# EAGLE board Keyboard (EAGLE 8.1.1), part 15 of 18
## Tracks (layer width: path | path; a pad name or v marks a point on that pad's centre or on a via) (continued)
S$15455 (continued)
  Bottom 0: 222.84,60.24 222.79,60.14
S$15456
  Bottom 0: 222.79,60.14 222.71,59.8
S$15457
  Bottom 0: 222.71,59.8 222.71,59.45
S$15458
  Bottom 0: 222.71,59.45 222.79,59.11
S$15459
  Bottom 0: 222.79,59.11 222.96,58.8
S$15460
  Bottom 0: 222.96,58.8 223.2,58.55
S$15461
  Bottom 0: 223.2,58.55 223.5,58.36
S$15462
  Bottom 0: 223.5,58.36 223.83,58.26
S$15463
  Bottom 0: 223.83,58.26 224.18,58.23
S$15464
  Bottom 0: 224.18,58.23 224.52,58.3
S$15465
  Bottom 0: 224.52,58.3 224.84,58.45
S$15466
  Bottom 0: 224.84,58.45 225.11,58.67
S$15467
  Bottom 0: 225.11,58.67 225.32,58.96
S$15468
  Bottom 0: 225.32,58.96 225.44,59.28
S$15469
  Bottom 0: 225.44,59.28 225.49,59.63
S$15470
  Bottom 0: 225.49,59.63 225.44,59.97
S$15471
  Bottom 0: 225.44,59.97 225.32,60.3
S$15472
  Bottom 0: 225.32,60.3 225.11,60.58
S$15473
  Bottom 0: 225.11,60.58 224.84,60.8
S$15474
  Bottom 0: 224.84,60.8 224.52,60.96
S$15475
  Bottom 0: 224.52,60.96 224.18,61.02
S$15476
  Bottom 0: 224.18,61.02 223.83,61
S$15477
  Bottom 0: 223.83,61 223.5,60.89
S$15478
  Bottom 0: 223.5,60.89 223.47,60.87
S$15479
  Bottom 0: 223.47,60.87 222.89,61.45
S$15480
  Bottom 0: 222.89,61.45 222.84,61.48
S$15481
  Bottom 0: 222.84,61.48 222.78,61.53
S$15482
  Bottom 0: 222.78,61.53 222.72,61.55
S$15483
  Bottom 0: 222.72,61.55 222.65,61.57
S$15484
  Bottom 0: 222.65,61.57 222.58,61.57
S$15485
  Bottom 0: 222.58,61.57 218.02,61.57
S$15486
  Bottom 0: 218.02,61.57 217.96,61.7
S$15487
  Bottom 0: 217.96,61.7 217.94,61.73
S$15488
  Bottom 0: 217.94,61.73 229.12,61.73
S$15489
  Bottom 0: 229.12,61.73 229.14,61.65
S$15490
  Bottom 0: 229.14,61.65 229.31,61.34
S$15491
  Bottom 0: 229.31,61.34 229.55,61.09
S$15492
  Bottom 0: 229.55,61.09 229.85,60.9
S$15493
  Bottom 0: 229.85,60.9 230.18,60.8
S$15494
  Bottom 0: 230.18,60.8 230.53,60.77
S$15495
  Bottom 0: 230.53,60.77 230.87,60.84
S$15496
  Bottom 0: 230.87,60.84 231.19,60.99
S$15497
  Bottom 0: 231.19,60.99 231.46,61.21
S$15498
  Bottom 0: 231.46,61.21 231.67,61.5
S$15499
  Bottom 0: 231.67,61.5 231.76,61.73
S$15500
  Bottom 0: 231.76,61.73 231.79,61.73
S$15501
  Bottom 0: 231.79,61.73 241.11,52.41
S$15502
  Bottom 0: 227.53,52.8 227.85,52.82
S$15503
  Bottom 0: 227.85,52.82 228.16,52.93
S$15504
  Bottom 0: 228.16,52.93 228.42,53.11
S$15505
  Bottom 0: 228.42,53.11 228.62,53.37
S$15506
  Bottom 0: 228.62,53.37 228.75,53.67
S$15507
  Bottom 0: 228.75,53.67 228.8,53.98
S$15508
  Bottom 0: 228.8,53.98 228.75,54.3
S$15509
  Bottom 0: 228.75,54.3 228.62,54.61
S$15510
  Bottom 0: 228.62,54.61 228.42,54.86
S$15511
  Bottom 0: 228.42,54.86 228.16,55.05
S$15512
  Bottom 0: 228.16,55.05 227.85,55.16
S$15513
  Bottom 0: 227.85,55.16 227.53,55.18
S$15514
  Bottom 0: 227.53,55.18 227.21,55.11
S$15515
  Bottom 0: 227.21,55.11 226.91,54.96
S$15516
  Bottom 0: 226.91,54.96 226.68,54.74
S$15517
  Bottom 0: 226.68,54.74 226.51,54.47
S$15518
  Bottom 0: 226.51,54.47 226.42,54.15
S$15519
  Bottom 0: 226.42,54.15 226.42,53.83
S$15520
  Bottom 0: 226.42,53.83 226.51,53.51
S$15521
  Bottom 0: 226.51,53.51 226.68,53.23
S$15522
  Bottom 0: 226.68,53.23 226.91,53.01
S$15523
  Bottom 0: 226.91,53.01 227.21,52.87
S$15524
  Bottom 0: 227.21,52.87 227.53,52.8
S$15525
  Bottom 0: 235.15,52.8 235.47,52.82
S$15526
  Bottom 0: 235.47,52.82 235.78,52.93
S$15527
  Bottom 0: 235.78,52.93 236.04,53.11
S$15528
  Bottom 0: 236.04,53.11 236.25,53.37
S$15529
  Bottom 0: 236.25,53.37 236.37,53.67
S$15530
  Bottom 0: 236.37,53.67 236.42,53.98
S$15531
  Bottom 0: 236.42,53.98 236.37,54.3
S$15532
  Bottom 0: 236.37,54.3 236.25,54.61
S$15533
  Bottom 0: 236.25,54.61 236.04,54.86
S$15534
  Bottom 0: 236.04,54.86 235.78,55.05
S$15535
  Bottom 0: 235.78,55.05 235.47,55.16
S$15536
  Bottom 0: 235.47,55.16 235.15,55.18
S$15537
  Bottom 0: 235.15,55.18 234.83,55.11
S$15538
  Bottom 0: 234.83,55.11 234.53,54.96
S$15539
  Bottom 0: 234.53,54.96 234.3,54.74
S$15540
  Bottom 0: 234.3,54.74 234.13,54.47
S$15541
  Bottom 0: 234.13,54.47 234.04,54.15
S$15542
  Bottom 0: 234.04,54.15 234.04,53.83
S$15543
  Bottom 0: 234.04,53.83 234.13,53.51
S$15544
  Bottom 0: 234.13,53.51 234.3,53.23
S$15545
  Bottom 0: 234.3,53.23 234.53,53.01
S$15546
  Bottom 0: 234.53,53.01 234.83,52.87
S$15547
  Bottom 0: 234.83,52.87 235.15,52.8
S$15548
  Bottom 0: 103.73,52.93 103,53.65
S$15549
  Bottom 0: 103,53.65 103.01,53.67
S$15550
  Bottom 0: 103.01,53.67 103.06,53.98
S$15551
  Bottom 0: 103.06,53.98 103.01,54.3
S$15552
  Bottom 0: 103.01,54.3 103,54.33
S$15553
  Bottom 0: 103,54.33 104.49,55.82
S$15554
  Bottom 0: 104.49,55.82 104.55,55.88
S$15555
  Bottom 0: 104.55,55.88 104.6,55.96
S$15556
  Bottom 0: 104.6,55.96 104.64,56.04
S$15557
  Bottom 0: 104.64,56.04 104.66,56.13
S$15558
  Bottom 0: 104.66,56.13 104.66,56.22
S$15559
  Bottom 0: 104.66,56.22 104.66,72.65
S$15560
  Bottom 0: 104.66,72.65 104.97,72.95
S$15561
  Bottom 0: 104.97,72.95 104.97,72.9
S$15562
  Bottom 0: 104.97,72.9 105.06,72.67
S$15563
  Bottom 0: 105.06,72.67 105.23,72.48
S$15564
  Bottom 0: 105.23,72.48 105.45,72.37
S$15565
  Bottom 0: 105.45,72.37 105.48,72.37
S$15566
  Bottom 0: 105.48,72.37 110.3,67.55
S$15567
  Bottom 0: 110.3,67.55 110.36,67.51
S$15568
  Bottom 0: 110.36,67.51 110.42,67.47
S$15569
  Bottom 0: 110.42,67.47 110.48,67.44
S$15570
  Bottom 0: 110.48,67.44 110.54,67.42
S$15571
  Bottom 0: 110.54,67.42 110.61,67.42
S$15572
  Bottom 0: 110.61,67.42 112.51,67.42
S$15573
  Bottom 0: 112.51,67.42 113.08,66.86
S$15574
  Bottom 0: 113.08,66.86 112.78,66.94
S$15575
  Bottom 0: 112.78,66.94 112.33,66.99
S$15576
  Bottom 0: 112.33,66.99 111.88,66.94
S$15577
  Bottom 0: 111.88,66.94 111.45,66.82
S$15578
  Bottom 0: 111.45,66.82 111.06,66.61
S$15579
  Bottom 0: 111.06,66.61 110.72,66.32
S$15580
  Bottom 0: 110.72,66.32 110.43,65.98
S$15581
  Bottom 0: 110.43,65.98 110.22,65.58
S$15582
  Bottom 0: 110.22,65.58 110.09,65.15
S$15583
  Bottom 0: 110.09,65.15 110.05,64.71
S$15584
  Bottom 0: 110.05,64.71 110.09,64.26
S$15585
  Bottom 0: 110.09,64.26 110.22,63.83
S$15586
  Bottom 0: 110.22,63.83 110.43,63.44
S$15587
  Bottom 0: 110.43,63.44 110.72,63.09
S$15588
  Bottom 0: 110.72,63.09 111.06,62.81
S$15589
  Bottom 0: 111.06,62.81 111.45,62.59
S$15590
  Bottom 0: 111.45,62.59 111.88,62.47
S$15591
  Bottom 0: 111.88,62.47 112.33,62.42
S$15592
  Bottom 0: 112.33,62.42 112.78,62.47
S$15593
  Bottom 0: 112.78,62.47 113.2,62.59
S$15594
  Bottom 0: 113.2,62.59 113.6,62.81
S$15595
  Bottom 0: 113.6,62.81 113.95,63.09
S$15596
  Bottom 0: 113.95,63.09 114.23,63.44
S$15597
  Bottom 0: 114.23,63.44 114.44,63.83
S$15598
  Bottom 0: 114.44,63.83 114.57,64.26
S$15599
  Bottom 0: 114.57,64.26 114.62,64.71
S$15600
  Bottom 0: 114.62,64.71 114.57,65.15
S$15601
  Bottom 0: 114.57,65.15 114.48,65.45
S$15602
  Bottom 0: 114.48,65.45 115.7,64.24
S$15603
  Bottom 0: 115.7,64.24 115.7,63.48
S$15604
  Bottom 0: 115.7,63.48 115.55,63.43
S$15605
  Bottom 0: 115.55,63.43 115.25,63.24
S$15606
  Bottom 0: 115.25,63.24 115.01,62.99
S$15607
  Bottom 0: 115.01,62.99 114.84,62.68
S$15608
  Bottom 0: 114.84,62.68 114.75,62.34
S$15609
  Bottom 0: 114.75,62.34 114.75,61.99
S$15610
  Bottom 0: 114.75,61.99 114.84,61.65
S$15611
  Bottom 0: 114.84,61.65 115.01,61.34
S$15612
  Bottom 0: 115.01,61.34 115.25,61.09
S$15613
  Bottom 0: 115.25,61.09 115.55,60.9
S$15614
  Bottom 0: 115.55,60.9 115.88,60.8
S$15615
  Bottom 0: 115.88,60.8 116.23,60.77
S$15616
  Bottom 0: 116.23,60.77 116.57,60.84
S$15617
  Bottom 0: 116.57,60.84 116.75,60.93
S$15618
  Bottom 0: 116.75,60.93 121.83,55.85
S$15619
  Bottom 0: 121.83,55.85 121.83,54.74
S$15620
  Bottom 0: 121.83,54.74 121.73,54.87
S$15621
  Bottom 0: 121.73,54.87 121.47,55.05
S$15622
  Bottom 0: 121.47,55.05 121.16,55.16
S$15623
  Bottom 0: 121.16,55.16 120.83,55.18
S$15624
  Bottom 0: 120.83,55.18 120.52,55.12
S$15625
  Bottom 0: 120.52,55.12 120.23,54.97
S$15626
  Bottom 0: 120.23,54.97 119.99,54.74
S$15627
  Bottom 0: 119.99,54.74 119.82,54.47
S$15628
  Bottom 0: 119.82,54.47 119.73,54.16
S$15629
  Bottom 0: 119.73,54.16 119.73,53.83
S$15630
  Bottom 0: 119.73,53.83 119.78,53.66
S$15631
  Bottom 0: 119.78,53.66 119.04,52.93
S$15632
  Bottom 0: 119.04,52.93 113.83,52.93
S$15633
  Bottom 0: 113.83,52.93 113.84,52.93
S$15634
  Bottom 0: 113.84,52.93 114.11,53.12
S$15635
  Bottom 0: 114.11,53.12 114.32,53.37
S$15636
  Bottom 0: 114.32,53.37 114.44,53.67
S$15637
  Bottom 0: 114.44,53.67 114.49,53.99
S$15638
  Bottom 0: 114.49,53.99 114.44,54.31
S$15639
  Bottom 0: 114.44,54.31 114.32,54.61
S$15640
  Bottom 0: 114.32,54.61 114.11,54.87
S$15641
  Bottom 0: 114.11,54.87 113.84,55.05
S$15642
  Bottom 0: 113.84,55.05 113.54,55.16
S$15643
  Bottom 0: 113.54,55.16 113.22,55.18
S$15644
  Bottom 0: 113.22,55.18 112.89,55.12
S$15645
  Bottom 0: 112.89,55.12 112.61,54.97
S$15646
  Bottom 0: 112.61,54.97 112.37,54.74
S$15647
  Bottom 0: 112.37,54.74 112.2,54.47
S$15648
  Bottom 0: 112.2,54.47 112.11,54.16
S$15649
  Bottom 0: 112.11,54.16 112.11,53.83
S$15650
  Bottom 0: 112.11,53.83 112.2,53.52
S$15651
  Bottom 0: 112.2,53.52 112.37,53.24
S$15652
  Bottom 0: 112.37,53.24 112.61,53.02
S$15653
  Bottom 0: 112.61,53.02 112.78,52.93
S$15654
  Bottom 0: 112.78,52.93 103.73,52.93
S$15655
  Bottom 0: 109.88,58.23 110.22,58.3
S$15656
  Bottom 0: 110.22,58.3 110.54,58.45
S$15657
  Bottom 0: 110.54,58.45 110.81,58.67
S$15658
  Bottom 0: 110.81,58.67 111.02,58.96
S$15659
  Bottom 0: 111.02,58.96 111.14,59.28
S$15660
  Bottom 0: 111.14,59.28 111.19,59.63
S$15661
  Bottom 0: 111.19,59.63 111.14,59.97
S$15662
  Bottom 0: 111.14,59.97 111.02,60.3
S$15663
  Bottom 0: 111.02,60.3 110.81,60.58
S$15664
  Bottom 0: 110.81,60.58 110.54,60.8
S$15665
  Bottom 0: 110.54,60.8 110.22,60.96
S$15666
  Bottom 0: 110.22,60.96 109.88,61.02
S$15667
  Bottom 0: 109.88,61.02 109.53,61
S$15668
  Bottom 0: 109.53,61 109.2,60.89
S$15669
  Bottom 0: 109.2,60.89 108.9,60.7
S$15670
  Bottom 0: 108.9,60.7 108.66,60.45
S$15671
  Bottom 0: 108.66,60.45 108.49,60.14
S$15672
  Bottom 0: 108.49,60.14 108.41,59.8
S$15673
  Bottom 0: 108.41,59.8 108.41,59.45
S$15674
  Bottom 0: 108.41,59.45 108.49,59.11
S$15675
  Bottom 0: 108.49,59.11 108.66,58.8
S$15676
  Bottom 0: 108.66,58.8 108.9,58.55
S$15677
  Bottom 0: 108.9,58.55 109.2,58.36
S$15678
  Bottom 0: 109.2,58.36 109.53,58.26
S$15679
  Bottom 0: 109.53,58.26 109.88,58.23
S$15680
  Bottom 0: 262.06,52.98 258.88,56.16
S$15681
  Bottom 0: 258.88,56.16 258.87,56.17
S$15682
  Bottom 0: 258.87,56.17 253.59,61.45
S$15683
  Bottom 0: 253.59,61.45 253.53,61.5
S$15684
  Bottom 0: 253.53,61.5 253.48,61.54
S$15685
  Bottom 0: 253.48,61.54 253.41,61.56
S$15686
  Bottom 0: 253.41,61.56 253.35,61.58
S$15687
  Bottom 0: 253.35,61.58 253.28,61.58
S$15688
  Bottom 0: 253.28,61.58 250.75,61.58
S$15689
  Bottom 0: 250.75,61.58 250.84,61.82
S$15690
  Bottom 0: 250.84,61.82 250.89,62.17
S$15691
  Bottom 0: 250.89,62.17 250.84,62.51
S$15692
  Bottom 0: 250.84,62.51 250.72,62.84
S$15693
  Bottom 0: 250.72,62.84 250.51,63.12
S$15694
  Bottom 0: 250.51,63.12 250.24,63.34
S$15695
  Bottom 0: 250.24,63.34 249.92,63.5
S$15696
  Bottom 0: 249.92,63.5 249.57,63.56
S$15697
  Bottom 0: 249.57,63.56 249.23,63.54
S$15698
  Bottom 0: 249.23,63.54 248.9,63.43
S$15699
  Bottom 0: 248.9,63.43 248.6,63.24
S$15700
  Bottom 0: 248.6,63.24 248.36,62.99
S$15701
  Bottom 0: 248.36,62.99 248.19,62.68
S$15702
  Bottom 0: 248.19,62.68 248.17,62.61
S$15703
  Bottom 0: 248.17,62.61 246.59,62.61
S$15704
  Bottom 0: 246.59,62.61 246.95,62.81
S$15705
  Bottom 0: 246.95,62.81 247.29,63.09
S$15706
  Bottom 0: 247.29,63.09 247.58,63.44
S$15707
  Bottom 0: 247.58,63.44 247.79,63.83
S$15708
  Bottom 0: 247.79,63.83 247.92,64.26
S$15709
  Bottom 0: 247.92,64.26 247.97,64.71
S$15710
  Bottom 0: 247.97,64.71 247.92,65.15
S$15711
  Bottom 0: 247.92,65.15 247.79,65.58
S$15712
  Bottom 0: 247.79,65.58 247.58,65.98
S$15713
  Bottom 0: 247.58,65.98 247.29,66.32
S$15714
  Bottom 0: 247.29,66.32 246.95,66.61
S$15715
  Bottom 0: 246.95,66.61 246.56,66.82
S$15716
  Bottom 0: 246.56,66.82 246.13,66.94
S$15717
  Bottom 0: 246.13,66.94 245.68,66.99
S$15718
  Bottom 0: 245.68,66.99 245.23,66.94
S$15719
  Bottom 0: 245.23,66.94 244.81,66.82
S$15720
  Bottom 0: 244.81,66.82 244.41,66.61
S$15721
  Bottom 0: 244.41,66.61 244.07,66.32
S$15722
  Bottom 0: 244.07,66.32 243.78,65.98
S$15723
  Bottom 0: 243.78,65.98 243.57,65.58
S$15724
  Bottom 0: 243.57,65.58 243.44,65.15
S$15725
  Bottom 0: 243.44,65.15 243.4,64.71
S$15726
  Bottom 0: 243.4,64.71 243.44,64.26
S$15727
  Bottom 0: 243.44,64.26 243.57,63.83
S$15728
  Bottom 0: 243.57,63.83 243.78,63.44
S$15729
  Bottom 0: 243.78,63.44 244.07,63.09
S$15730
  Bottom 0: 244.07,63.09 244.41,62.81
S$15731
  Bottom 0: 244.41,62.81 244.78,62.61
S$15732
  Bottom 0: 244.78,62.61 241.81,62.61
S$15733
  Bottom 0: 241.81,62.61 236.24,68.18
S$15734
  Bottom 0: 236.24,68.18 236.18,68.21
S$15735
  Bottom 0: 236.18,68.21 236.13,68.26
S$15736
  Bottom 0: 236.13,68.26 236.06,68.28
S$15737
  Bottom 0: 236.06,68.28 236,68.3
S$15738
  Bottom 0: 236,68.3 235.93,68.3
S$15739
  Bottom 0: 235.93,68.3 219.79,68.3
S$15740
  Bottom 0: 219.79,68.3 213.97,74.13
S$15741
  Bottom 0: 213.97,74.13 213.92,74.18
S$15742
  Bottom 0: 213.92,74.18 213.86,74.22
S$15743
  Bottom 0: 213.86,74.22 213.79,74.24
S$15744
  Bottom 0: 213.79,74.24 213.73,74.26
S$15745
  Bottom 0: 213.73,74.26 213.66,74.26
S$15746
  Bottom 0: 213.66,74.26 213.61,74.26
S$15747
  Bottom 0: 213.61,74.26 213.87,74.35
S$15748
  Bottom 0: 213.87,74.35 214.13,74.54
S$15749
  Bottom 0: 214.13,74.54 214.34,74.8
S$15750
  Bottom 0: 214.34,74.8 214.46,75.09
S$15751
  Bottom 0: 214.46,75.09 214.51,75.42
S$15752
  Bottom 0: 214.51,75.42 214.46,75.73
S$15753
  Bottom 0: 214.46,75.73 214.34,76.03
S$15754
  Bottom 0: 214.34,76.03 214.13,76.29
S$15755
  Bottom 0: 214.13,76.29 213.87,76.48
S$15756
  Bottom 0: 213.87,76.48 213.56,76.58
S$15757
  Bottom 0: 213.56,76.58 213.44,76.59
S$15758
  Bottom 0: 213.44,76.59 213.44,77.85
S$15759
  Bottom 0: 213.44,77.85 213.68,77.6
S$15760
  Bottom 0: 213.68,77.6 213.97,77.41
S$15761
  Bottom 0: 213.97,77.41 214.3,77.31
S$15762
  Bottom 0: 214.3,77.31 214.65,77.28
S$15763
  Bottom 0: 214.65,77.28 215,77.35
S$15764
  Bottom 0: 215,77.35 215.31,77.5
S$15765
  Bottom 0: 215.31,77.5 215.58,77.72
S$15766
  Bottom 0: 215.58,77.72 215.79,78.01
S$15767
  Bottom 0: 215.79,78.01 215.92,78.33
S$15768
  Bottom 0: 215.92,78.33 215.96,78.68
S$15769
  Bottom 0: 215.96,78.68 215.92,79.02
S$15770
  Bottom 0: 215.92,79.02 215.79,79.35
S$15771
  Bottom 0: 215.79,79.35 215.58,79.63
S$15772
  Bottom 0: 215.58,79.63 215.31,79.86
S$15773
  Bottom 0: 215.31,79.86 215.01,80
S$15774
  Bottom 0: 215.01,80 215.01,82.85
S$15775
  Bottom 0: 215.01,82.85 215.21,82.49
S$15776
  Bottom 0: 215.21,82.49 215.49,82.14
S$15777
  Bottom 0: 215.49,82.14 215.84,81.86
S$15778
  Bottom 0: 215.84,81.86 216.23,81.64
S$15779
  Bottom 0: 216.23,81.64 216.66,81.52
S$15780
  Bottom 0: 216.66,81.52 217.11,81.47
S$15781
  Bottom 0: 217.11,81.47 217.55,81.52
S$15782
  Bottom 0: 217.55,81.52 217.98,81.64
S$15783
  Bottom 0: 217.98,81.64 218.38,81.86
S$15784
  Bottom 0: 218.38,81.86 218.65,82.08
S$15785
  Bottom 0: 218.65,82.08 218.65,80.59
S$15786
  Bottom 0: 218.65,80.59 218.65,80.5
S$15787
  Bottom 0: 218.65,80.5 218.68,80.41
S$15788
  Bottom 0: 218.68,80.41 218.71,80.33
S$15789
  Bottom 0: 218.71,80.33 218.76,80.25
S$15790
  Bottom 0: 218.76,80.25 218.82,80.19
S$15791
  Bottom 0: 218.82,80.19 227.33,71.67
S$15792
  Bottom 0: 227.33,71.67 227.33,70.77
S$15793
  Bottom 0: 227.33,70.77 227.16,70.65
S$15794
  Bottom 0: 227.16,70.65 226.94,70.41
S$15795
  Bottom 0: 226.94,70.41 226.8,70.11
S$15796
  Bottom 0: 226.8,70.11 226.76,69.79
S$15797
  Bottom 0: 226.76,69.79 226.8,69.47
S$15798
  Bottom 0: 226.8,69.47 226.94,69.16
S$15799
  Bottom 0: 226.94,69.16 227.16,68.92
S$15800
  Bottom 0: 227.16,68.92 227.43,68.75
S$15801
  Bottom 0: 227.43,68.75 227.74,68.65
S$15802
  Bottom 0: 227.74,68.65 228.06,68.65
S$15803
  Bottom 0: 228.06,68.65 228.37,68.75
S$15804
  Bottom 0: 228.37,68.75 228.65,68.92
S$15805
  Bottom 0: 228.65,68.92 228.86,69.16
S$15806
  Bottom 0: 228.86,69.16 229,69.47
S$15807
  Bottom 0: 229,69.47 229.04,69.79
S$15808
  Bottom 0: 229.04,69.79 229,70.11
S$15809
  Bottom 0: 229,70.11 228.86,70.41
S$15810
  Bottom 0: 228.86,70.41 228.65,70.65
S$15811
  Bottom 0: 228.65,70.65 228.47,70.77
S$15812
  Bottom 0: 228.47,70.77 228.47,71.91
S$15813
  Bottom 0: 228.47,71.91 228.47,72
S$15814
  Bottom 0: 228.47,72 228.44,72.08
S$15815
  Bottom 0: 228.44,72.08 228.41,72.16
S$15816
  Bottom 0: 228.41,72.16 228.36,72.24
S$15817
  Bottom 0: 228.36,72.24 228.3,72.3
S$15818
  Bottom 0: 228.3,72.3 220.77,79.84
S$15819
  Bottom 0: 220.77,79.84 221,79.83
S$15820
  Bottom 0: 221,79.83 221.35,79.89
S$15821
  Bottom 0: 221.35,79.89 221.53,79.97
S$15822
  Bottom 0: 221.53,79.97 222.84,78.66
S$15823
  Bottom 0: 222.84,78.66 222.9,78.62
S$15824
  Bottom 0: 222.9,78.62 222.95,78.58
S$15825
  Bottom 0: 222.95,78.58 223.02,78.55
S$15826
  Bottom 0: 223.02,78.55 223.09,78.53
S$15827
  Bottom 0: 223.09,78.53 223.16,78.53
S$15828
  Bottom 0: 223.16,78.53 226.2,78.53
S$15829
  Bottom 0: 226.2,78.53 230.51,74.22
S$15830
  Bottom 0: 230.51,74.22 230.38,74.23
S$15831
  Bottom 0: 230.38,74.23 230.06,74.17
S$15832
  Bottom 0: 230.06,74.17 229.77,74.02
S$15833
  Bottom 0: 229.77,74.02 229.54,73.8
S$15834
  Bottom 0: 229.54,73.8 229.37,73.52
S$15835
  Bottom 0: 229.37,73.52 229.28,73.2
S$15836
  Bottom 0: 229.28,73.2 229.28,72.88
S$15837
  Bottom 0: 229.28,72.88 229.37,72.56
S$15838
  Bottom 0: 229.37,72.56 229.54,72.29
S$15839
  Bottom 0: 229.54,72.29 229.77,72.07
S$15840
  Bottom 0: 229.77,72.07 230.06,71.92
S$15841
  Bottom 0: 230.06,71.92 230.38,71.85
S$15842
  Bottom 0: 230.38,71.85 230.71,71.87
S$15843
  Bottom 0: 230.71,71.87 231.01,71.98
S$15844
  Bottom 0: 231.01,71.98 231.28,72.17
S$15845
  Bottom 0: 231.28,72.17 231.48,72.42
S$15846
  Bottom 0: 231.48,72.42 231.61,72.72
S$15847
  Bottom 0: 231.61,72.72 231.66,73.04
S$15848
  Bottom 0: 231.66,73.04 231.65,73.08
S$15849
  Bottom 0: 231.65,73.08 237.29,67.44
S$15850
  Bottom 0: 237.29,67.44 237.34,67.4
S$15851
  Bottom 0: 237.34,67.4 237.41,67.36
S$15852
  Bottom 0: 237.41,67.36 237.47,67.33
S$15853
  Bottom 0: 237.47,67.33 237.53,67.32
S$15854
  Bottom 0: 237.53,67.32 237.6,67.31
S$15855
  Bottom 0: 237.6,67.31 246.94,67.31
S$15856
  Bottom 0: 246.94,67.31 252.4,61.85
S$15857
  Bottom 0: 252.4,61.85 252.45,61.81
S$15858
  Bottom 0: 252.45,61.81 252.51,61.77
S$15859
  Bottom 0: 252.51,61.77 252.57,61.74
S$15860
  Bottom 0: 252.57,61.74 252.64,61.73
S$15861
  Bottom 0: 252.64,61.73 252.71,61.73
S$15862
  Bottom 0: 252.71,61.73 271.98,61.73
S$15863
  Bottom 0: 271.98,61.73 272,61.65
S$15864
  Bottom 0: 272,61.65 272.17,61.34
S$15865
  Bottom 0: 272.17,61.34 272.41,61.09
S$15866
  Bottom 0: 272.41,61.09 272.71,60.9
S$15867
  Bottom 0: 272.71,60.9 273.04,60.8
S$15868
  Bottom 0: 273.04,60.8 273.39,60.77
S$15869
  Bottom 0: 273.39,60.77 273.73,60.84
S$15870
  Bottom 0: 273.73,60.84 274.05,60.99
S$15871
  Bottom 0: 274.05,60.99 274.32,61.21
S$15872
  Bottom 0: 274.32,61.21 274.53,61.5
S$15873
  Bottom 0: 274.53,61.5 274.65,61.82
S$15874
  Bottom 0: 274.65,61.82 274.7,62.17
S$15875
  Bottom 0: 274.7,62.17 274.65,62.51
S$15876
  Bottom 0: 274.65,62.51 274.53,62.84
S$15877
  Bottom 0: 274.53,62.84 274.32,63.12
S$15878
  Bottom 0: 274.32,63.12 274.05,63.34
S$15879
  Bottom 0: 274.05,63.34 273.73,63.5
S$15880
  Bottom 0: 273.73,63.5 273.39,63.56
S$15881
  Bottom 0: 273.39,63.56 273.04,63.54
S$15882
  Bottom 0: 273.04,63.54 272.71,63.43
S$15883
  Bottom 0: 272.71,63.43 272.41,63.24
S$15884
  Bottom 0: 272.41,63.24 272.17,62.99
S$15885
  Bottom 0: 272.17,62.99 272,62.68
S$15886
  Bottom 0: 272,62.68 271.98,62.61
S$15887
  Bottom 0: 271.98,62.61 270.4,62.61
S$15888
  Bottom 0: 270.4,62.61 270.76,62.81
S$15889
  Bottom 0: 270.76,62.81 271.1,63.09
S$15890
  Bottom 0: 271.1,63.09 271.39,63.44
S$15891
  Bottom 0: 271.39,63.44 271.61,63.83
S$15892
  Bottom 0: 271.61,63.83 271.73,64.26
S$15893
  Bottom 0: 271.73,64.26 271.78,64.71
S$15894
  Bottom 0: 271.78,64.71 271.73,65.15
S$15895
  Bottom 0: 271.73,65.15 271.61,65.58
S$15896
  Bottom 0: 271.61,65.58 271.39,65.98
S$15897
  Bottom 0: 271.39,65.98 271.1,66.32
S$15898
  Bottom 0: 271.1,66.32 270.76,66.61
S$15899
  Bottom 0: 270.76,66.61 270.46,66.77
S$15900
  Bottom 0: 270.46,66.77 273.35,66.77
S$15901
  Bottom 0: 273.35,66.77 278.05,62.07
S$15902
  Bottom 0: 278.05,62.07 277.77,62.09
S$15903
  Bottom 0: 277.77,62.09 277.45,62.02
S$15904
  Bottom 0: 277.45,62.02 277.17,61.87
S$15905
  Bottom 0: 277.17,61.87 276.93,61.65
S$15906
  Bottom 0: 276.93,61.65 276.76,61.37
S$15907
  Bottom 0: 276.76,61.37 276.68,61.06
S$15908
  Bottom 0: 276.68,61.06 276.68,60.73
S$15909
  Bottom 0: 276.68,60.73 276.72,60.56
S$15910
  Bottom 0: 276.72,60.56 270.72,54.56
S$15911
  Bottom 0: 270.72,54.56 267.23,54.56
S$15912
  Bottom 0: 267.23,54.56 267.21,54.61
S$15913
  Bottom 0: 267.21,54.61 267,54.87
S$15914
  Bottom 0: 267,54.87 266.74,55.05
S$15915
  Bottom 0: 266.74,55.05 266.43,55.16
S$15916
  Bottom 0: 266.43,55.16 266.11,55.18
S$15917
  Bottom 0: 266.11,55.18 265.79,55.12
S$15918
  Bottom 0: 265.79,55.12 265.5,54.97
S$15919
  Bottom 0: 265.5,54.97 265.26,54.74
S$15920
  Bottom 0: 265.26,54.74 265.09,54.47
S$15921
  Bottom 0: 265.09,54.47 265.01,54.16
S$15922
  Bottom 0: 265.01,54.16 265.01,53.83
S$15923
  Bottom 0: 265.01,53.83 265.09,53.52
S$15924
  Bottom 0: 265.09,53.52 265.26,53.24
S$15925
  Bottom 0: 265.26,53.24 265.5,53.02
S$15926
  Bottom 0: 265.5,53.02 265.57,52.98
S$15927
  Bottom 0: 265.57,52.98 262.06,52.98
S$15928
  Bottom 0: 261.26,57.74 261.56,57.81
S$15929
  Bottom 0: 261.56,57.81 261.82,57.96
S$15930
  Bottom 0: 261.82,57.96 262.02,58.18
S$15931
  Bottom 0: 262.02,58.18 262.15,58.45
S$15932
  Bottom 0: 262.15,58.45 262.2,58.75
S$15933
  Bottom 0: 262.2,58.75 262.15,59.05
S$15934
  Bottom 0: 262.15,59.05 262.02,59.32
S$15935
  Bottom 0: 262.02,59.32 261.82,59.55
S$15936
  Bottom 0: 261.82,59.55 261.56,59.7
S$15937
  Bottom 0: 261.56,59.7 261.26,59.76
S$15938
  Bottom 0: 261.26,59.76 260.96,59.74
S$15939
  Bottom 0: 260.96,59.74 260.68,59.63
S$15940
  Bottom 0: 260.68,59.63 260.44,59.44
S$15941
  Bottom 0: 260.44,59.44 260.27,59.19
S$15942
  Bottom 0: 260.27,59.19 260.18,58.91
S$15943
  Bottom 0: 260.18,58.91 260.18,58.6
S$15944
  Bottom 0: 260.18,58.6 260.27,58.31
S$15945
  Bottom 0: 260.27,58.31 260.44,58.06
S$15946
  Bottom 0: 260.44,58.06 260.68,57.87
S$15947
  Bottom 0: 260.68,57.87 260.96,57.76
S$15948
  Bottom 0: 260.96,57.76 261.26,57.74
S$15949
  Bottom 0: 267.04,58.23 267.38,58.3
S$15950
  Bottom 0: 267.38,58.3 267.7,58.45
S$15951
  Bottom 0: 267.7,58.45 267.97,58.67
S$15952
  Bottom 0: 267.97,58.67 268.18,58.96
S$15953
  Bottom 0: 268.18,58.96 268.3,59.28
S$15954
  Bottom 0: 268.3,59.28 268.35,59.63
S$15955
  Bottom 0: 268.35,59.63 268.3,59.97
S$15956
  Bottom 0: 268.3,59.97 268.18,60.3
S$15957
  Bottom 0: 268.18,60.3 267.97,60.58
S$15958
  Bottom 0: 267.97,60.58 267.7,60.8
S$15959
  Bottom 0: 267.7,60.8 267.38,60.96
S$15960
  Bottom 0: 267.38,60.96 267.04,61.02
S$15961
  Bottom 0: 267.04,61.02 266.69,61
S$15962
  Bottom 0: 266.69,61 266.36,60.89
S$15963
  Bottom 0: 266.36,60.89 266.06,60.7
S$15964
  Bottom 0: 266.06,60.7 265.82,60.45
S$15965
  Bottom 0: 265.82,60.45 265.65,60.14
S$15966
  Bottom 0: 265.65,60.14 265.56,59.8
S$15967
  Bottom 0: 265.56,59.8 265.56,59.45
S$15968
  Bottom 0: 265.56,59.45 265.65,59.11
S$15969
  Bottom 0: 265.65,59.11 265.82,58.8
S$15970
  Bottom 0: 265.82,58.8 266.06,58.55
S$15971
  Bottom 0: 266.06,58.55 266.36,58.36
S$15972
  Bottom 0: 266.36,58.36 266.69,58.26
S$15973
  Bottom 0: 266.69,58.26 267.04,58.23
S$15974
  Bottom 0: 257.69,59.65 257.98,59.71
S$15975
  Bottom 0: 257.98,59.71 258.24,59.87
S$15976
  Bottom 0: 258.24,59.87 258.45,60.08
S$15977
  Bottom 0: 258.45,60.08 258.58,60.36
S$15978
  Bottom 0: 258.58,60.36 258.62,60.66
S$15979
  Bottom 0: 258.62,60.66 258.58,60.96
S$15980
  Bottom 0: 258.58,60.96 258.45,61.23
S$15981
  Bottom 0: 258.45,61.23 258.24,61.45
S$15982
  Bottom 0: 258.24,61.45 257.98,61.6
S$15983
  Bottom 0: 257.98,61.6 257.69,61.67
S$15984
  Bottom 0: 257.69,61.67 257.38,61.65
S$15985
  Bottom 0: 257.38,61.65 257.1,61.54
S$15986
  Bottom 0: 257.1,61.54 256.86,61.35
S$15987
  Bottom 0: 256.86,61.35 256.69,61.1
S$15988
  Bottom 0: 256.69,61.1 256.6,60.81
S$15989
  Bottom 0: 256.6,60.81 256.6,60.51
S$15990
  Bottom 0: 256.6,60.51 256.69,60.21
S$15991
  Bottom 0: 256.69,60.21 256.86,59.97
S$15992
  Bottom 0: 256.86,59.97 257.1,59.78
S$15993
  Bottom 0: 257.1,59.78 257.38,59.67
S$15994
  Bottom 0: 257.38,59.67 257.69,59.65
S$15995
  Bottom 0: 224.47,68.64 226.25,68.64
S$15996
  Bottom 0: 226.25,68.64 226.33,68.65
S$15997
  Bottom 0: 226.33,68.65 226.4,68.69
S$15998
  Bottom 0: 226.4,68.69 226.45,68.75
S$15999
  Bottom 0: 226.45,68.75 226.49,68.82
S$16000
  Bottom 0: 226.49,68.82 226.5,68.9
S$16001
  Bottom 0: 226.5,68.9 226.5,70.67
S$16002
  Bottom 0: 226.5,70.67 226.49,70.75
S$16003
  Bottom 0: 226.49,70.75 226.45,70.82
S$16004
  Bottom 0: 226.45,70.82 226.4,70.88
S$16005
  Bottom 0: 226.4,70.88 226.33,70.92
S$16006
  Bottom 0: 226.33,70.92 226.25,70.93
S$16007
  Bottom 0: 226.25,70.93 225.8,70.93
S$16008
  Bottom 0: 225.8,70.93 225.8,71.06
S$16009
  Bottom 0: 225.8,71.06 225.74,71.28
S$16010
  Bottom 0: 225.74,71.28 225.58,71.44
S$16011
  Bottom 0: 225.58,71.44 225.36,71.5
S$16012
  Bottom 0: 225.36,71.5 225.02,71.5
S$16013
  Bottom 0: 225.02,71.5 223.93,72.58
S$16014
  Bottom 0: 223.93,72.58 223.99,72.72
S$16015
  Bottom 0: 223.99,72.72 224.04,73.04
S$16016
  Bottom 0: 224.04,73.04 223.99,73.36
S$16017
  Bottom 0: 223.99,73.36 223.86,73.66
S$16018
  Bottom 0: 223.86,73.66 223.66,73.92
S$16019
  Bottom 0: 223.66,73.92 223.39,74.11
S$16020
  Bottom 0: 223.39,74.11 223.09,74.21
S$16021
  Bottom 0: 223.09,74.21 222.76,74.23
S$16022
  Bottom 0: 222.76,74.23 222.44,74.17
S$16023
  Bottom 0: 222.44,74.17 222.15,74.02
S$16024
  Bottom 0: 222.15,74.02 221.92,73.8
S$16025
  Bottom 0: 221.92,73.8 221.75,73.52
S$16026
  Bottom 0: 221.75,73.52 221.66,73.2
S$16027
  Bottom 0: 221.66,73.2 221.66,72.88
S$16028
  Bottom 0: 221.66,72.88 221.75,72.56
S$16029
  Bottom 0: 221.75,72.56 221.92,72.29
S$16030
  Bottom 0: 221.92,72.29 222.15,72.07
S$16031
  Bottom 0: 222.15,72.07 222.44,71.92
S$16032
  Bottom 0: 222.44,71.92 222.76,71.85
S$16033
  Bottom 0: 222.76,71.85 223.09,71.87
S$16034
  Bottom 0: 223.09,71.87 223.31,71.95
S$16035
  Bottom 0: 223.31,71.95 224.37,70.9
S$16036
  Bottom 0: 224.37,70.9 224.32,70.88
S$16037
  Bottom 0: 224.32,70.88 224.27,70.82
S$16038
  Bottom 0: 224.27,70.82 224.23,70.75
S$16039
  Bottom 0: 224.23,70.75 224.22,70.67
S$16040
  Bottom 0: 224.22,70.67 224.22,68.9
S$16041
  Bottom 0: 224.22,68.9 224.23,68.82
S$16042
  Bottom 0: 224.23,68.82 224.27,68.75
S$16043
  Bottom 0: 224.27,68.75 224.32,68.69
S$16044
  Bottom 0: 224.32,68.69 224.4,68.65
S$16045
  Bottom 0: 224.4,68.65 224.47,68.64
S$16046
  Bottom 0: 220.86,74.23 221.18,74.24
S$16047
  Bottom 0: 221.18,74.24 221.49,74.35
S$16048
  Bottom 0: 221.49,74.35 221.75,74.54
S$16049
  Bottom 0: 221.75,74.54 221.96,74.8
S$16050
  Bottom 0: 221.96,74.8 222.08,75.09
S$16051
  Bottom 0: 222.08,75.09 222.13,75.42
S$16052
  Bottom 0: 222.13,75.42 222.08,75.73
S$16053
  Bottom 0: 222.08,75.73 221.96,76.03
S$16054
  Bottom 0: 221.96,76.03 221.75,76.29
S$16055
  Bottom 0: 221.75,76.29 221.49,76.48
S$16056
  Bottom 0: 221.49,76.48 221.18,76.58
S$16057
  Bottom 0: 221.18,76.58 220.86,76.6
S$16058
  Bottom 0: 220.86,76.6 220.54,76.54
S$16059
  Bottom 0: 220.54,76.54 220.24,76.39
S$16060
  Bottom 0: 220.24,76.39 220.01,76.17
S$16061
  Bottom 0: 220.01,76.17 219.84,75.89
S$16062
  Bottom 0: 219.84,75.89 219.75,75.58
S$16063
  Bottom 0: 219.75,75.58 219.75,75.25
S$16064
  Bottom 0: 219.75,75.25 219.84,74.94
S$16065
  Bottom 0: 219.84,74.94 220.01,74.66
S$16066
  Bottom 0: 220.01,74.66 220.24,74.44
S$16067
  Bottom 0: 220.24,74.44 220.54,74.29
S$16068
  Bottom 0: 220.54,74.29 220.86,74.23
S$16069
  Bottom 0: 41.18,54.81 33.38,62.62
S$16070
  Bottom 0: 33.38,62.62 33.32,62.66
S$16071
  Bottom 0: 33.32,62.66 33.26,62.7
S$16072
  Bottom 0: 33.26,62.7 33.2,62.73
S$16073
  Bottom 0: 33.2,62.73 33.13,62.75
S$16074
  Bottom 0: 33.13,62.75 33.06,62.75
S$16075
  Bottom 0: 33.06,62.75 31.55,62.75
S$16076
  Bottom 0: 31.55,62.75 31.55,63.18
S$16077
  Bottom 0: 31.55,63.18 31.54,63.25
S$16078
  Bottom 0: 31.54,63.25 31.53,63.32
S$16079
  Bottom 0: 31.53,63.32 31.5,63.38
S$16080
  Bottom 0: 31.5,63.38 31.46,63.44
S$16081
  Bottom 0: 31.46,63.44 31.42,63.5
S$16082
  Bottom 0: 31.42,63.5 30.95,63.97
S$16083
  Bottom 0: 30.95,63.97 30.9,64
S$16084
  Bottom 0: 30.9,64 30.84,64.05
S$16085
  Bottom 0: 30.84,64.05 30.78,64.07
S$16086
  Bottom 0: 30.78,64.07 30.71,64.08
S$16087
  Bottom 0: 30.71,64.08 30.64,64.09
S$16088
  Bottom 0: 30.64,64.09 30.14,64.09
S$16089
  Bottom 0: 30.14,64.09 26.48,67.76
S$16090
  Bottom 0: 26.48,67.76 26.68,67.74
S$16091
  Bottom 0: 26.68,67.74 26.98,67.81
S$16092
  Bottom 0: 26.98,67.81 27.24,67.96
S$16093
  Bottom 0: 27.24,67.96 27.25,67.97
S$16094
  Bottom 0: 27.25,67.97 37.98,67.97
S$16095
  Bottom 0: 37.98,67.97 38.05,67.98
S$16096
  Bottom 0: 38.05,67.98 38.12,67.99
S$16097
  Bottom 0: 38.12,67.99 38.18,68.02
S$16098
  Bottom 0: 38.18,68.02 38.24,68.06
S$16099
  Bottom 0: 38.24,68.06 38.29,68.1
S$16100
  Bottom 0: 38.29,68.1 39.63,69.44
S$16101
  Bottom 0: 39.63,69.44 44.91,69.44
S$16102
  Bottom 0: 44.91,69.44 44.74,69.19
S$16103
  Bottom 0: 44.74,69.19 44.65,68.9
S$16104
  Bottom 0: 44.65,68.9 44.65,68.59
S$16105
  Bottom 0: 44.65,68.59 44.74,68.31
S$16106
  Bottom 0: 44.74,68.31 44.91,68.06
S$16107
  Bottom 0: 44.91,68.06 45.15,67.87
S$16108
  Bottom 0: 45.15,67.87 45.43,67.76
S$16109
  Bottom 0: 45.43,67.76 45.73,67.74
S$16110
  Bottom 0: 45.73,67.74 45.98,67.8
S$16111
  Bottom 0: 45.98,67.8 46.2,67.57
S$16112
  Bottom 0: 46.2,67.57 46.22,67.56
S$16113
  Bottom 0: 46.22,67.56 44.89,67.56
S$16114
  Bottom 0: 44.89,67.56 44.82,67.56
S$16115
  Bottom 0: 44.82,67.56 44.75,67.54
S$16116
  Bottom 0: 44.75,67.54 44.68,67.51
S$16117
  Bottom 0: 44.68,67.51 44.63,67.47
S$16118
  Bottom 0: 44.63,67.47 44.57,67.43
S$16119
  Bottom 0: 44.57,67.43 40.55,63.41
S$16120
  Bottom 0: 40.55,63.41 40.37,63.5
S$16121
  Bottom 0: 40.37,63.5 40.03,63.56
S$16122
  Bottom 0: 40.03,63.56 39.68,63.54
S$16123
  Bottom 0: 39.68,63.54 39.34,63.43
S$16124
  Bottom 0: 39.34,63.43 39.05,63.24
S$16125
  Bottom 0: 39.05,63.24 38.81,62.99
S$16126
  Bottom 0: 38.81,62.99 38.64,62.68
S$16127
  Bottom 0: 38.64,62.68 38.55,62.34
S$16128
  Bottom 0: 38.55,62.34 38.55,61.99
S$16129
  Bottom 0: 38.55,61.99 38.64,61.65
S$16130
  Bottom 0: 38.64,61.65 38.81,61.34
S$16131
  Bottom 0: 38.81,61.34 39.05,61.09
S$16132
  Bottom 0: 39.05,61.09 39.34,60.9
S$16133
  Bottom 0: 39.34,60.9 39.68,60.8
S$16134
  Bottom 0: 39.68,60.8 40.03,60.77
S$16135
  Bottom 0: 40.03,60.77 40.37,60.84
S$16136
  Bottom 0: 40.37,60.84 40.69,60.99
S$16137
  Bottom 0: 40.69,60.99 40.96,61.21
S$16138
  Bottom 0: 40.96,61.21 41.17,61.5
S$16139
  Bottom 0: 41.17,61.5 41.29,61.82
S$16140
  Bottom 0: 41.29,61.82 41.34,62.17
S$16141
  Bottom 0: 41.34,62.17 41.29,62.51
S$16142
  Bottom 0: 41.29,62.51 41.18,62.79
S$16143
  Bottom 0: 41.18,62.79 45.07,66.68
S$16144
  Bottom 0: 45.07,66.68 54.04,66.68
S$16145
  Bottom 0: 54.04,66.68 53.91,66.61
S$16146
  Bottom 0: 53.91,66.61 53.57,66.32
S$16147
  Bottom 0: 53.57,66.32 53.28,65.98
S$16148
  Bottom 0: 53.28,65.98 53.07,65.58
S$16149
  Bottom 0: 53.07,65.58 52.94,65.15
S$16150
  Bottom 0: 52.94,65.15 52.9,64.71
S$16151
  Bottom 0: 52.9,64.71 52.94,64.26
S$16152
  Bottom 0: 52.94,64.26 53.07,63.83
S$16153
  Bottom 0: 53.07,63.83 53.28,63.44
S$16154
  Bottom 0: 53.28,63.44 53.57,63.09
S$16155
  Bottom 0: 53.57,63.09 53.91,62.81
S$16156
  Bottom 0: 53.91,62.81 54.3,62.59
S$16157
  Bottom 0: 54.3,62.59 54.73,62.47
S$16158
  Bottom 0: 54.73,62.47 55.18,62.42
S$16159
  Bottom 0: 55.18,62.42 55.63,62.47
S$16160
  Bottom 0: 55.63,62.47 56.05,62.59
S$16161
  Bottom 0: 56.05,62.59 56.45,62.81
S$16162
  Bottom 0: 56.45,62.81 56.8,63.09
S$16163
  Bottom 0: 56.8,63.09 57.08,63.44
S$16164
  Bottom 0: 57.08,63.44 57.3,63.83
S$16165
  Bottom 0: 57.3,63.83 57.42,64.26
S$16166
  Bottom 0: 57.42,64.26 57.47,64.71
S$16167
  Bottom 0: 57.47,64.71 57.42,65.15
S$16168
  Bottom 0: 57.42,65.15 57.3,65.58
S$16169
  Bottom 0: 57.3,65.58 57.08,65.98
S$16170
  Bottom 0: 57.08,65.98 56.8,66.32
S$16171
  Bottom 0: 56.8,66.32 56.45,66.61
S$16172
  Bottom 0: 56.45,66.61 56.32,66.68
S$16173
  Bottom 0: 56.32,66.68 73.09,66.68
S$16174
  Bottom 0: 73.09,66.68 72.96,66.61
S$16175
  Bottom 0: 72.96,66.61 72.62,66.32
S$16176
  Bottom 0: 72.62,66.32 72.33,65.98
S$16177
  Bottom 0: 72.33,65.98 72.12,65.58
S$16178
  Bottom 0: 72.12,65.58 71.99,65.15
S$16179
  Bottom 0: 71.99,65.15 71.94,64.71
S$16180
  Bottom 0: 71.94,64.71 71.99,64.26
S$16181
  Bottom 0: 71.99,64.26 72.12,63.83
S$16182
  Bottom 0: 72.12,63.83 72.33,63.44
S$16183
  Bottom 0: 72.33,63.44 72.62,63.09
S$16184
  Bottom 0: 72.62,63.09 72.96,62.81
S$16185
  Bottom 0: 72.96,62.81 73.36,62.59
S$16186
  Bottom 0: 73.36,62.59 73.78,62.47
S$16187
  Bottom 0: 73.78,62.47 74.23,62.42
S$16188
  Bottom 0: 74.23,62.42 74.68,62.47
S$16189
  Bottom 0: 74.68,62.47 75.11,62.59
S$16190
  Bottom 0: 75.11,62.59 75.5,62.81
S$16191
  Bottom 0: 75.5,62.81 75.85,63.09
S$16192
  Bottom 0: 75.85,63.09 76.13,63.44
S$16193
  Bottom 0: 76.13,63.44 76.34,63.83
S$16194
  Bottom 0: 76.34,63.83 76.47,64.26
S$16195
  Bottom 0: 76.47,64.26 76.52,64.71
S$16196
  Bottom 0: 76.52,64.71 76.47,65.15
S$16197
  Bottom 0: 76.47,65.15 76.43,65.28
S$16198
  Bottom 0: 76.43,65.28 78.16,63.55
S$16199
  Bottom 0: 78.16,63.55 78.13,63.56
S$16200
  Bottom 0: 78.13,63.56 77.78,63.54
S$16201
  Bottom 0: 77.78,63.54 77.44,63.43
S$16202
  Bottom 0: 77.44,63.43 77.15,63.24
S$16203
  Bottom 0: 77.15,63.24 76.91,62.99
S$16204
  Bottom 0: 76.91,62.99 76.74,62.68
S$16205
  Bottom 0: 76.74,62.68 76.65,62.34
S$16206
  Bottom 0: 76.65,62.34 76.65,61.99
S$16207
  Bottom 0: 76.65,61.99 76.74,61.65
S$16208
  Bottom 0: 76.74,61.65 76.8,61.55
S$16209
  Bottom 0: 76.8,61.55 74.2,58.96
S$16210
  Bottom 0: 74.2,58.96 74.16,58.9
S$16211
  Bottom 0: 74.16,58.9 74.12,58.84
S$16212
  Bottom 0: 74.12,58.84 74.09,58.78
S$16213
  Bottom 0: 74.09,58.78 74.08,58.71
S$16214
  Bottom 0: 74.08,58.71 74.07,58.64
S$16215
  Bottom 0: 74.07,58.64 74.07,58.58
S$16216
  Bottom 0: 74.07,58.58 72.21,56.72
S$16217
  Bottom 0: 72.21,56.72 43.28,56.72
S$16218
  Bottom 0: 43.28,56.72 43.21,56.72
S$16219
  Bottom 0: 43.21,56.72 43.14,56.7
S$16220
  Bottom 0: 43.14,56.7 43.08,56.67
S$16221
  Bottom 0: 43.08,56.67 43.02,56.63
S$16222
  Bottom 0: 43.02,56.63 42.96,56.59
S$16223
  Bottom 0: 42.96,56.59 41.18,54.81
S$16224
  Bottom 0: 71.78,58.23 72.12,58.3
S$16225
  Bottom 0: 72.12,58.3 72.44,58.45
S$16226
  Bottom 0: 72.44,58.45 72.71,58.67
S$16227
  Bottom 0: 72.71,58.67 72.92,58.96
S$16228
  Bottom 0: 72.92,58.96 73.04,59.28
S$16229
  Bottom 0: 73.04,59.28 73.09,59.63
S$16230
  Bottom 0: 73.09,59.63 73.04,59.97
S$16231
  Bottom 0: 73.04,59.97 72.92,60.3
S$16232
  Bottom 0: 72.92,60.3 72.71,60.58
S$16233
  Bottom 0: 72.71,60.58 72.44,60.8
S$16234
  Bottom 0: 72.44,60.8 72.12,60.96
S$16235
  Bottom 0: 72.12,60.96 71.78,61.02
S$16236
  Bottom 0: 71.78,61.02 71.43,61
S$16237
  Bottom 0: 71.43,61 71.09,60.89
S$16238
  Bottom 0: 71.09,60.89 71.06,60.87
S$16239
  Bottom 0: 71.06,60.87 70.49,61.45
S$16240
  Bottom 0: 70.49,61.45 70.44,61.48
S$16241
  Bottom 0: 70.44,61.48 70.38,61.53
S$16242
  Bottom 0: 70.38,61.53 70.32,61.55
S$16243
  Bottom 0: 70.32,61.55 70.25,61.57
S$16244
  Bottom 0: 70.25,61.57 70.18,61.57
S$16245
  Bottom 0: 70.18,61.57 65.61,61.57
S$16246
  Bottom 0: 65.61,61.57 65.54,61.7
S$16247
  Bottom 0: 65.54,61.7 65.34,61.92
S$16248
  Bottom 0: 65.34,61.92 65.08,62.08
S$16249
  Bottom 0: 65.08,62.08 64.78,62.14
S$16250
  Bottom 0: 64.78,62.14 64.48,62.12
S$16251
  Bottom 0: 64.48,62.12 64.2,62.01
S$16252
  Bottom 0: 64.2,62.01 63.96,61.82
S$16253
  Bottom 0: 63.96,61.82 63.79,61.57
S$16254
  Bottom 0: 63.79,61.57 63.7,61.28
S$16255
  Bottom 0: 63.7,61.28 63.7,60.98
S$16256
  Bottom 0: 63.7,60.98 63.79,60.69
S$16257
  Bottom 0: 63.79,60.69 63.96,60.44
S$16258
  Bottom 0: 63.96,60.44 64.2,60.25
S$16259
  Bottom 0: 64.2,60.25 64.48,60.14
S$16260
  Bottom 0: 64.48,60.14 64.78,60.12
S$16261
  Bottom 0: 64.78,60.12 65.08,60.19
S$16262
  Bottom 0: 65.08,60.19 65.34,60.34
S$16263
  Bottom 0: 65.34,60.34 65.54,60.56
S$16264
  Bottom 0: 65.54,60.56 65.61,60.69
S$16265
  Bottom 0: 65.61,60.69 70,60.69
S$16266
  Bottom 0: 70,60.69 70.45,60.24
S$16267
  Bottom 0: 70.45,60.24 70.39,60.14
S$16268
  Bottom 0: 70.39,60.14 70.3,59.8
S$16269
  Bottom 0: 70.3,59.8 70.3,59.45
S$16270
  Bottom 0: 70.3,59.45 70.39,59.11
S$16271
  Bottom 0: 70.39,59.11 70.56,58.8
S$16272
  Bottom 0: 70.56,58.8 70.8,58.55
S$16273
  Bottom 0: 70.8,58.55 71.09,58.36
S$16274
  Bottom 0: 71.09,58.36 71.43,58.26
S$16275
  Bottom 0: 71.43,58.26 71.78,58.23
S$16276
  Bottom 0: 52.73,58.23 53.07,58.3
S$16277
  Bottom 0: 53.07,58.3 53.39,58.45
S$16278
  Bottom 0: 53.39,58.45 53.66,58.67
S$16279
  Bottom 0: 53.66,58.67 53.87,58.96
S$16280
  Bottom 0: 53.87,58.96 53.99,59.28
S$16281
  Bottom 0: 53.99,59.28 54.04,59.63
S$16282
  Bottom 0: 54.04,59.63 53.99,59.97
S$16283
  Bottom 0: 53.99,59.97 53.87,60.3
S$16284
  Bottom 0: 53.87,60.3 53.66,60.58
S$16285
  Bottom 0: 53.66,60.58 53.39,60.8
S$16286
  Bottom 0: 53.39,60.8 53.07,60.96
S$16287
  Bottom 0: 53.07,60.96 52.73,61.02
S$16288
  Bottom 0: 52.73,61.02 52.38,61
S$16289
  Bottom 0: 52.38,61 52.05,60.89
S$16290
  Bottom 0: 52.05,60.89 52.02,60.87
S$16291
  Bottom 0: 52.02,60.87 51.45,61.45
S$16292
  Bottom 0: 51.45,61.45 51.4,61.48
S$16293
  Bottom 0: 51.4,61.48 51.34,61.53
S$16294
  Bottom 0: 51.34,61.53 51.27,61.55
S$16295
  Bottom 0: 51.27,61.55 51.21,61.57
S$16296
  Bottom 0: 51.21,61.57 51.14,61.57
S$16297
  Bottom 0: 51.14,61.57 46.56,61.57
S$16298
  Bottom 0: 46.56,61.57 46.49,61.7
S$16299
  Bottom 0: 46.49,61.7 46.29,61.92
S$16300
  Bottom 0: 46.29,61.92 46.03,62.08
S$16301
  Bottom 0: 46.03,62.08 45.73,62.14
S$16302
  Bottom 0: 45.73,62.14 45.43,62.12
S$16303
  Bottom 0: 45.43,62.12 45.15,62.01
S$16304
  Bottom 0: 45.15,62.01 44.91,61.82
S$16305
  Bottom 0: 44.91,61.82 44.74,61.57
S$16306
  Bottom 0: 44.74,61.57 44.65,61.28
S$16307
  Bottom 0: 44.65,61.28 44.65,60.98
S$16308
  Bottom 0: 44.65,60.98 44.74,60.69
S$16309
  Bottom 0: 44.74,60.69 44.91,60.44
S$16310
  Bottom 0: 44.91,60.44 45.15,60.25
S$16311
  Bottom 0: 45.15,60.25 45.43,60.14
S$16312
  Bottom 0: 45.43,60.14 45.73,60.12
S$16313
  Bottom 0: 45.73,60.12 46.03,60.19
S$16314
  Bottom 0: 46.03,60.19 46.29,60.34
S$16315
  Bottom 0: 46.29,60.34 46.49,60.56
S$16316
  Bottom 0: 46.49,60.56 46.56,60.69
S$16317
  Bottom 0: 46.56,60.69 50.95,60.69
S$16318
  Bottom 0: 50.95,60.69 51.4,60.24
S$16319
  Bottom 0: 51.4,60.24 51.34,60.14
S$16320
  Bottom 0: 51.34,60.14 51.25,59.8
S$16321
  Bottom 0: 51.25,59.8 51.25,59.45
S$16322
  Bottom 0: 51.25,59.45 51.34,59.11
S$16323
  Bottom 0: 51.34,59.11 51.51,58.8
S$16324
  Bottom 0: 51.51,58.8 51.75,58.55
S$16325
  Bottom 0: 51.75,58.55 52.05,58.36
S$16326
  Bottom 0: 52.05,58.36 52.38,58.26
S$16327
  Bottom 0: 52.38,58.26 52.73,58.23
S$16328
  Bottom 0: 59.08,60.77 59.42,60.84
S$16329
  Bottom 0: 59.42,60.84 59.74,60.99
S$16330
  Bottom 0: 59.74,60.99 60.01,61.21
S$16331
  Bottom 0: 60.01,61.21 60.22,61.5
S$16332
  Bottom 0: 60.22,61.5 60.34,61.82
S$16333
  Bottom 0: 60.34,61.82 60.39,62.17
S$16334
  Bottom 0: 60.39,62.17 60.34,62.51
S$16335
  Bottom 0: 60.34,62.51 60.22,62.84
S$16336
  Bottom 0: 60.22,62.84 60.01,63.12
S$16337
  Bottom 0: 60.01,63.12 59.74,63.34
S$16338
  Bottom 0: 59.74,63.34 59.42,63.5
S$16339
  Bottom 0: 59.42,63.5 59.08,63.56
S$16340
  Bottom 0: 59.08,63.56 58.73,63.54
S$16341
  Bottom 0: 58.73,63.54 58.4,63.43
S$16342
  Bottom 0: 58.4,63.43 58.1,63.24
S$16343
  Bottom 0: 58.1,63.24 57.86,62.99
S$16344
  Bottom 0: 57.86,62.99 57.69,62.68
S$16345
  Bottom 0: 57.69,62.68 57.6,62.34
S$16346
  Bottom 0: 57.6,62.34 57.6,61.99
S$16347
  Bottom 0: 57.6,61.99 57.69,61.65
S$16348
  Bottom 0: 57.69,61.65 57.86,61.34
S$16349
  Bottom 0: 57.86,61.34 58.1,61.09
S$16350
  Bottom 0: 58.1,61.09 58.4,60.9
S$16351
  Bottom 0: 58.4,60.9 58.73,60.8
S$16352
  Bottom 0: 58.73,60.8 59.08,60.77
S$16353
  Bottom 0: 36.13,62.42 36.58,62.47
S$16354
  Bottom 0: 36.58,62.47 37.01,62.59
S$16355
  Bottom 0: 37.01,62.59 37.4,62.81
S$16356
  Bottom 0: 37.4,62.81 37.75,63.09
S$16357
  Bottom 0: 37.75,63.09 38.03,63.44
S$16358
  Bottom 0: 38.03,63.44 38.24,63.83
S$16359
  Bottom 0: 38.24,63.83 38.37,64.26
S$16360
  Bottom 0: 38.37,64.26 38.42,64.71
S$16361
  Bottom 0: 38.42,64.71 38.37,65.15
S$16362
  Bottom 0: 38.37,65.15 38.24,65.58
S$16363
  Bottom 0: 38.24,65.58 38.03,65.98
S$16364
  Bottom 0: 38.03,65.98 37.75,66.32
S$16365
  Bottom 0: 37.75,66.32 37.4,66.61
S$16366
  Bottom 0: 37.4,66.61 37.01,66.82
S$16367
  Bottom 0: 37.01,66.82 36.58,66.94
S$16368
  Bottom 0: 36.58,66.94 36.13,66.99
S$16369
  Bottom 0: 36.13,66.99 35.68,66.94
S$16370
  Bottom 0: 35.68,66.94 35.26,66.82
S$16371
  Bottom 0: 35.26,66.82 34.86,66.61
S$16372
  Bottom 0: 34.86,66.61 34.51,66.32
S$16373
  Bottom 0: 34.51,66.32 34.23,65.98
S$16374
  Bottom 0: 34.23,65.98 34.02,65.58
S$16375
  Bottom 0: 34.02,65.58 33.89,65.15
S$16376
  Bottom 0: 33.89,65.15 33.85,64.71
S$16377
  Bottom 0: 33.85,64.71 33.89,64.26
S$16378
  Bottom 0: 33.89,64.26 34.02,63.83
S$16379
  Bottom 0: 34.02,63.83 34.23,63.44
S$16380
  Bottom 0: 34.23,63.44 34.51,63.09
S$16381
  Bottom 0: 34.51,63.09 34.86,62.81
S$16382
  Bottom 0: 34.86,62.81 35.26,62.59
S$16383
  Bottom 0: 35.26,62.59 35.68,62.47
S$16384
  Bottom 0: 35.68,62.47 36.13,62.42
S$16385
  Bottom 0: 316.02,54.84 309.66,61.21
S$16386
  Bottom 0: 309.66,61.21 309.66,66.88
S$16387
  Bottom 0: 309.66,66.88 316.02,60.52
S$16388
  Bottom 0: 316.02,60.52 316.02,54.84
S$16389
  Bottom 0: 313.89,58.22 314.19,58.27
S$16390
  Bottom 0: 314.19,58.27 314.3,58.24
S$16391
  Bottom 0: 314.3,58.24 314.65,58.22
S$16392
  Bottom 0: 314.65,58.22 315,58.28
S$16393
  Bottom 0: 315,58.28 315.31,58.43
S$16394
  Bottom 0: 315.31,58.43 315.58,58.66
S$16395
  Bottom 0: 315.58,58.66 315.79,58.94
S$16396
  Bottom 0: 315.79,58.94 315.92,59.27
S$16397
  Bottom 0: 315.92,59.27 315.96,59.61
S$16398
  Bottom 0: 315.96,59.61 315.92,59.95
S$16399
  Bottom 0: 315.92,59.95 315.79,60.28
S$16400
  Bottom 0: 315.79,60.28 315.58,60.57
S$16401
  Bottom 0: 315.58,60.57 315.31,60.79
S$16402
  Bottom 0: 315.31,60.79 315,60.94
S$16403
  Bottom 0: 315,60.94 314.65,61
S$16404
  Bottom 0: 314.65,61 314.3,60.98
S$16405
  Bottom 0: 314.3,60.98 314.19,60.95
S$16406
  Bottom 0: 314.19,60.95 313.89,61
S$16407
  Bottom 0: 313.89,61 313.54,60.98
S$16408
  Bottom 0: 313.54,60.98 313.21,60.87
S$16409
  Bottom 0: 313.21,60.87 312.92,60.69
S$16410
  Bottom 0: 312.92,60.69 312.68,60.43
S$16411
  Bottom 0: 312.68,60.43 312.5,60.12
S$16412
  Bottom 0: 312.5,60.12 312.42,59.78
S$16413
  Bottom 0: 312.42,59.78 312.42,59.44
S$16414
  Bottom 0: 312.42,59.44 312.5,59.1
S$16415
  Bottom 0: 312.5,59.1 312.68,58.79
S$16416
  Bottom 0: 312.68,58.79 312.92,58.53
S$16417
  Bottom 0: 312.92,58.53 313.21,58.35
S$16418
  Bottom 0: 313.21,58.35 313.54,58.24
S$16419
  Bottom 0: 313.54,58.24 313.89,58.22
S$16420
  Bottom 0: 149.76,54.93 149.76,56.27
S$16421
  Bottom 0: 149.76,56.27 154.27,60.78
S$16422
  Bottom 0: 154.27,60.78 154.33,60.77
S$16423
  Bottom 0: 154.33,60.77 154.67,60.84
S$16424
  Bottom 0: 154.67,60.84 154.99,60.99
S$16425
  Bottom 0: 154.99,60.99 155.26,61.21
S$16426
  Bottom 0: 155.26,61.21 155.47,61.5
S$16427
  Bottom 0: 155.47,61.5 155.59,61.82
S$16428
  Bottom 0: 155.59,61.82 155.64,62.17
S$16429
  Bottom 0: 155.64,62.17 155.59,62.51
S$16430
  Bottom 0: 155.59,62.51 155.47,62.84
S$16431
  Bottom 0: 155.47,62.84 155.26,63.12
S$16432
  Bottom 0: 155.26,63.12 155,63.34
S$16433
  Bottom 0: 155,63.34 155,68.87
S$16434
  Bottom 0: 155,68.87 157.2,66.67
S$16435
  Bottom 0: 157.2,66.67 157.2,63.25
S$16436
  Bottom 0: 157.2,63.25 157.06,63.11
S$16437
  Bottom 0: 157.06,63.11 156.97,62.87
S$16438
  Bottom 0: 156.97,62.87 156.97,62.62
S$16439
  Bottom 0: 156.97,62.62 157.06,62.38
S$16440
  Bottom 0: 157.06,62.38 157.13,62.3
S$16441
  Bottom 0: 157.13,62.3 157.08,62.26
S$16442
  Bottom 0: 157.08,62.26 149.77,54.96
S$16443
  Bottom 0: 149.77,54.96 149.76,54.93
S$16444
  Bottom 0: 316.72,61.07 310.22,67.57
S$16445
  Bottom 0: 310.22,67.57 310.22,68.43
S$16446
  Bottom 0: 310.22,68.43 310.21,68.5
S$16447
  Bottom 0: 310.21,68.5 310.2,68.57
S$16448
  Bottom 0: 310.2,68.57 310.17,68.63
S$16449
  Bottom 0: 310.17,68.63 310.13,68.69
S$16450
  Bottom 0: 310.13,68.69 310.09,68.75
S$16451
  Bottom 0: 310.09,68.75 308.73,70.1
S$16452
  Bottom 0: 308.73,70.1 309.25,70.1
S$16453
  Bottom 0: 309.25,70.1 311.25,68.09
S$16454
  Bottom 0: 311.25,68.09 311.31,68.05
S$16455
  Bottom 0: 311.31,68.05 311.37,68.01
S$16456
  Bottom 0: 311.37,68.01 311.43,67.99
S$16457
  Bottom 0: 311.43,67.99 311.5,67.97
S$16458
  Bottom 0: 311.5,67.97 311.57,67.97
S$16459
  Bottom 0: 311.57,67.97 318.94,67.97
S$16460
  Bottom 0: 318.94,67.97 319.01,67.97
S$16461
  Bottom 0: 319.01,67.97 319.08,67.99
S$16462
  Bottom 0: 319.08,67.99 319.14,68.01
S$16463
  Bottom 0: 319.14,68.01 319.2,68.05
S$16464
  Bottom 0: 319.2,68.05 319.25,68.09
S$16465
  Bottom 0: 319.25,68.09 319.97,68.81
S$16466
  Bottom 0: 319.97,68.81 320,68.86
S$16467
  Bottom 0: 320,68.86 320.05,68.92
S$16468
  Bottom 0: 320.05,68.92 320.07,68.98
S$16469
  Bottom 0: 320.07,68.98 320.09,69.05
S$16470
  Bottom 0: 320.09,69.05 320.09,69.12
S$16471
  Bottom 0: 320.09,69.12 320.09,72.23
S$16472
  Bottom 0: 320.09,72.23 320.27,72.07
S$16473
  Bottom 0: 320.27,72.07 320.56,71.92
S$16474
  Bottom 0: 320.56,71.92 320.88,71.85
S$16475
  Bottom 0: 320.88,71.85 321.2,71.87
S$16476
  Bottom 0: 321.2,71.87 321.51,71.98
S$16477
  Bottom 0: 321.51,71.98 321.77,72.17
S$16478
  Bottom 0: 321.77,72.17 321.98,72.42
S$16479
  Bottom 0: 321.98,72.42 322.05,72.58
S$16480
  Bottom 0: 322.05,72.58 322.05,66.83
S$16481
  Bottom 0: 322.05,66.83 319.29,64.07
S$16482
  Bottom 0: 319.29,64.07 319.34,64.24
S$16483
  Bottom 0: 319.34,64.24 319.39,64.69
S$16484
  Bottom 0: 319.39,64.69 319.34,65.14
S$16485
  Bottom 0: 319.34,65.14 319.21,65.56
S$16486
  Bottom 0: 319.21,65.56 319,65.96
S$16487
  Bottom 0: 319,65.96 318.72,66.3
S$16488
  Bottom 0: 318.72,66.3 318.37,66.59
S$16489
  Bottom 0: 318.37,66.59 317.97,66.81
S$16490
  Bottom 0: 317.97,66.81 317.55,66.93
S$16491
  Bottom 0: 317.55,66.93 317.1,66.98
S$16492
  Bottom 0: 317.1,66.98 316.72,66.94
S$16493
  Bottom 0: 316.72,66.94 316.34,66.98
S$16494
  Bottom 0: 316.34,66.98 315.89,66.93
S$16495
  Bottom 0: 315.89,66.93 315.46,66.81
S$16496
  Bottom 0: 315.46,66.81 315.07,66.59
S$16497
  Bottom 0: 315.07,66.59 314.72,66.3
S$16498
  Bottom 0: 314.72,66.3 314.44,65.96
S$16499
  Bottom 0: 314.44,65.96 314.22,65.56
S$16500
  Bottom 0: 314.22,65.56 314.1,65.14
S$16501
  Bottom 0: 314.1,65.14 314.05,64.69
S$16502
  Bottom 0: 314.05,64.69 314.1,64.24
S$16503
  Bottom 0: 314.1,64.24 314.22,63.82
S$16504
  Bottom 0: 314.22,63.82 314.44,63.42
S$16505
  Bottom 0: 314.44,63.42 314.72,63.08
S$16506
  Bottom 0: 314.72,63.08 315.07,62.79
S$16507
  Bottom 0: 315.07,62.79 315.46,62.58
S$16508
  Bottom 0: 315.46,62.58 315.89,62.45
S$16509
  Bottom 0: 315.89,62.45 316.34,62.41
S$16510
  Bottom 0: 316.34,62.41 316.72,62.45
S$16511
  Bottom 0: 316.72,62.45 317.1,62.41
S$16512
  Bottom 0: 317.1,62.41 317.55,62.45
S$16513
  Bottom 0: 317.55,62.45 317.72,62.5
S$16514
  Bottom 0: 317.72,62.5 316.85,61.63
S$16515
  Bottom 0: 316.85,61.63 316.81,61.58
S$16516
  Bottom 0: 316.81,61.58 316.76,61.52
S$16517
  Bottom 0: 316.76,61.52 316.74,61.45
S$16518
  Bottom 0: 316.74,61.45 316.73,61.39
S$16519
  Bottom 0: 316.73,61.39 316.72,61.32
S$16520
  Bottom 0: 316.72,61.32 316.72,61.07
S$16521
  Bottom 0: 254.76,62.61 254.84,62.73
S$16522
  Bottom 0: 254.84,62.73 254.88,62.98
S$16523
  Bottom 0: 254.88,62.98 254.84,63.23
S$16524
  Bottom 0: 254.84,63.23 254.7,63.44
S$16525
  Bottom 0: 254.7,63.44 254.5,63.59
S$16526
  Bottom 0: 254.5,63.59 254.26,63.66
S$16527
  Bottom 0: 254.26,63.66 254.15,63.65
S$16528
  Bottom 0: 254.15,63.65 249.16,68.64
S$16529
  Bottom 0: 249.16,68.64 249.1,68.68
S$16530
  Bottom 0: 249.1,68.68 249.04,68.72
S$16531
  Bottom 0: 249.04,68.72 248.98,68.75
S$16532
  Bottom 0: 248.98,68.75 248.92,68.77
S$16533
  Bottom 0: 248.92,68.77 248.85,68.77
S$16534
  Bottom 0: 248.85,68.77 247.47,68.77
S$16535
  Bottom 0: 247.47,68.77 247.7,68.92
S$16536
  Bottom 0: 247.7,68.92 247.91,69.16
S$16537
  Bottom 0: 247.91,69.16 248.05,69.47
S$16538
  Bottom 0: 248.05,69.47 248.09,69.79
S$16539
  Bottom 0: 248.09,69.79 248.05,70.11
S$16540
  Bottom 0: 248.05,70.11 247.91,70.41
S$16541
  Bottom 0: 247.91,70.41 247.7,70.65
S$16542
  Bottom 0: 247.7,70.65 247.42,70.83
S$16543
  Bottom 0: 247.42,70.83 247.11,70.92
S$16544
  Bottom 0: 247.11,70.92 246.79,70.92
S$16545
  Bottom 0: 246.79,70.92 246.48,70.83
S$16546
  Bottom 0: 246.48,70.83 246.21,70.65
S$16547
  Bottom 0: 246.21,70.65 246.12,70.56
S$16548
  Bottom 0: 246.12,70.56 246.12,72.05
S$16549
  Bottom 0: 246.12,72.05 246.12,72.12
S$16550
  Bottom 0: 246.12,72.12 246.1,72.19
S$16551
  Bottom 0: 246.1,72.19 246.08,72.25
S$16552
  Bottom 0: 246.08,72.25 246.04,72.31
S$16553
  Bottom 0: 246.04,72.31 246,72.37
S$16554
  Bottom 0: 246,72.37 238.83,79.53
S$16555
  Bottom 0: 238.83,79.53 238.83,80.4
S$16556
  Bottom 0: 238.83,80.4 238.84,80.39
S$16557
  Bottom 0: 238.84,80.39 239.08,80.14
S$16558
  Bottom 0: 239.08,80.14 239.37,79.95
S$16559
  Bottom 0: 239.37,79.95 239.7,79.84
S$16560
  Bottom 0: 239.7,79.84 240.03,79.83
S$16561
